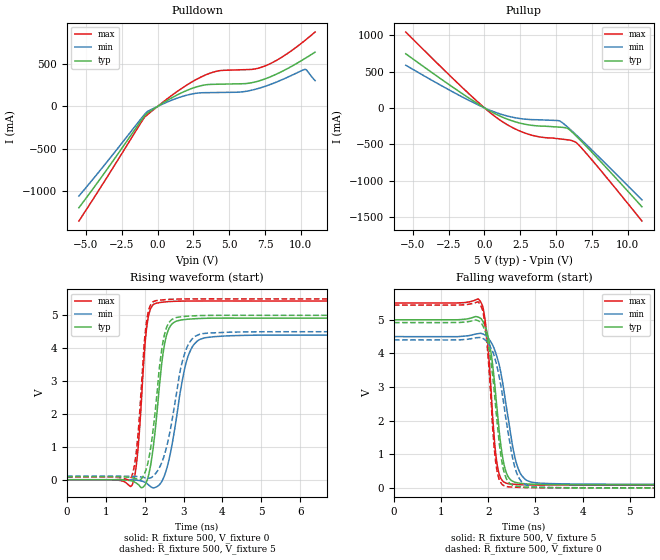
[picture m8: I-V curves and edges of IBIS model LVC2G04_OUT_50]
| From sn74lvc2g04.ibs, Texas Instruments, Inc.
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[Model]   LVC2G04_OUT_50
Model_type  Output
Vref =   0
Rref =   500
Cref =   50p
Vmeas =   2.5
| variable   typ   min   max
C_comp   8.88pF   5.46pF   12.35pF
| C_pullup   9.78pF   5.46pF   12.35pF
| C_pulldown   7.99pF   5.90pF   11.08pF
[Temperature Range]   40   100   -40
| Ambient temperature   25   85   -40
[Voltage range]   5   4.5   5.5
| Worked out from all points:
|   slope of the pulldown table from 0 to 0.75 V, typ, clamps not added: 9.58 ohm
|   slope of the pullup table from 0 to 0.75 V, typ, clamps not added: 9.16 ohm
|   rising waveform, R_fixture 500, V_fixture 0: 20-80 % time 265ps typ, 383ps min, 187ps max; typ from 0 V to 4.91 V
|   falling waveform, R_fixture 500, V_fixture 5: 20-80 % time 228ps typ, 314ps min, 167ps max; typ from 5 V to 0.09 V
|   rising waveform, R_fixture 500, V_fixture 5: 20-80 % time 279ps typ, 413ps min, 198ps max; typ from 0.09 V to 5 V
|   falling waveform, R_fixture 500, V_fixture 0: 20-80 % time 228ps typ, 318ps min, 165ps max; typ from 4.92 V to 0 V
[Pulldown]
| LVC2G04_OUT_50
|   Voltage   I(typ)   I(min)   I(max)
-5.5V     -1.198A    -1.059A    -1.354A
-970mV    -125.1mA   -106.1mA   -141.7mA
-675mV    -74.35mA   -56.48mA   -92.74mA
205mV     22.29mA    16.59mA    27.99mA
1.905V    179.2mA    127mA      238mA
3.285V    253.2mA    162.4mA    367.3mA
4.325V    262.7mA    164.8mA    422.2mA
5.815V    267.8mA    170.7mA    433mA
7.31V     313.8mA    226.4mA    466mA
8.65V     410.1mA    312.7mA    578.8mA
10.28V    565mA      437.4mA    777.7mA
11V       641.2mA    305.2mA    879.1mA
[Pullup]
| LVC2G04_OUT_50
|   Voltage   I(typ)   I(min)   I(max)
-5.5V     745.2mA    587.5mA    1.044A
-1.18V    147.6mA    112.6mA    211.7mA
170mV     -19.98mA   -14.91mA   -29.14mA
1.04V     -109.2mA   -79.97mA   -161.6mA
2.045V    -185.4mA   -131.8mA   -280mA
3.05V     -232.7mA   -158.7mA   -361.3mA
3.945V    -250.5mA   -165.3mA   -402.5mA
5.3V      -265.9mA   -185.4mA   -427.7mA
5.83V     -285.1mA   -268.2mA   -440mA
6.525V    -410.2mA   -394.3mA   -498.1mA
8.085V    -732.8mA   -692.6mA   -852.4mA
11V       -1.361A    -1.267A    -1.557A
[Ramp]
| LVC2G04_OUT_50
| variable   typ   min   max
dV/dt_r   3.09/2.87E-10   2.79/4.13E-10   3.39/2.01E-10
dV/dt_f   3.01/2.40E-10   2.69/3.30E-10   3.33/1.78E-10
R_load = 500
[Rising Waveform]
| LVC2G04_OUT_50
R_fixture =   500
C_fixture =   0
L_fixture =   0
V_fixture =   0
V_fixture_min = 0
V_fixture_max = 0
|   Time   V(typ)   V(min)   V(max)
0s        181.8pV    4.248nV    2.638nV
1.68ns    -39.4mV    -5.823mV   -145.2mV
1.82ns    -133.1mV   -17.77mV   853.5mV
2.06ns    -19.57mV   -118.2mV   4.713V
2.315ns   2.034V     -208.9mV   5.375V
2.465ns   3.788V     9.312mV    5.4V
2.625ns   4.603V     613.6mV    5.418V
3.09ns    4.88V      3.663V     5.434V
3.575ns   4.91V      4.322V     5.436V
24.99ns   4.914V     4.397V     5.435V
[Falling Waveform]
| LVC2G04_OUT_50
R_fixture =   500
C_fixture =   0
L_fixture =   0
V_fixture =   5
V_fixture_min = 4.5
V_fixture_max = 5.5
|   Time   V(typ)   V(min)   V(max)
0s        5V         4.5V       5.5V
1.835ns   5.048V     4.597V     5.54V
1.975ns   4.628V     4.495V     4.488V
2.075ns   3.859V     4.295V     2.547V
2.185ns   2.373V     3.896V     729.6mV
2.305ns   908.5mV    3.132V     207.1mV
2.435ns   305.8mV    1.966V     121.3mV
2.675ns   136.4mV    444.7mV    95.57mV
3.095ns   100.4mV    138.1mV    82.39mV
24.99ns   89.64mV    107.6mV    78.98mV
[Rising Waveform]
| LVC2G04_OUT_50
R_fixture =   500
C_fixture =   0
L_fixture =   0
V_fixture =   5
V_fixture_min = 4.5
V_fixture_max = 5.5
|   Time   V(typ)   V(min)   V(max)
0s        89.62mV    107.6mV    78.96mV
1.65ns    65.34mV    105.1mV    65.71mV
1.8ns     23.55mV    98.62mV    1.042V
2.05ns    374.6mV    54.13mV    4.83V
2.3ns     2.438V     220.9mV    5.449V
2.445ns   4.018V     543.1mV    5.467V
2.6ns     4.732V     1.181V     5.483V
3.01ns    4.966V     3.771V     5.498V
3.47ns    4.994V     4.44V      5.5V
24.99ns   5V         4.5V       5.5V
[Falling Waveform]
| LVC2G04_OUT_50
R_fixture =   500
C_fixture =   0
L_fixture =   0
V_fixture =   0
V_fixture_min = 0
V_fixture_max = 0
|   Time   V(typ)   V(min)   V(max)
0s        4.917V     4.401V     5.437V
1.82ns    4.945V     4.473V     5.472V
1.96ns    4.542V     4.367V     4.471V
2.065ns   3.659V     4.138V     2.477V
2.175ns   2.132V     3.672V     594.5mV
2.285ns   811.4mV    2.893V     116.7mV
2.41ns    204.6mV    1.746V     33.21mV
2.655ns   38.55mV    286.9mV    14.43mV
3.08ns    8.554mV    20.17mV    3.073mV
24.99ns   19.19uV    19.91uV    18.34uV
